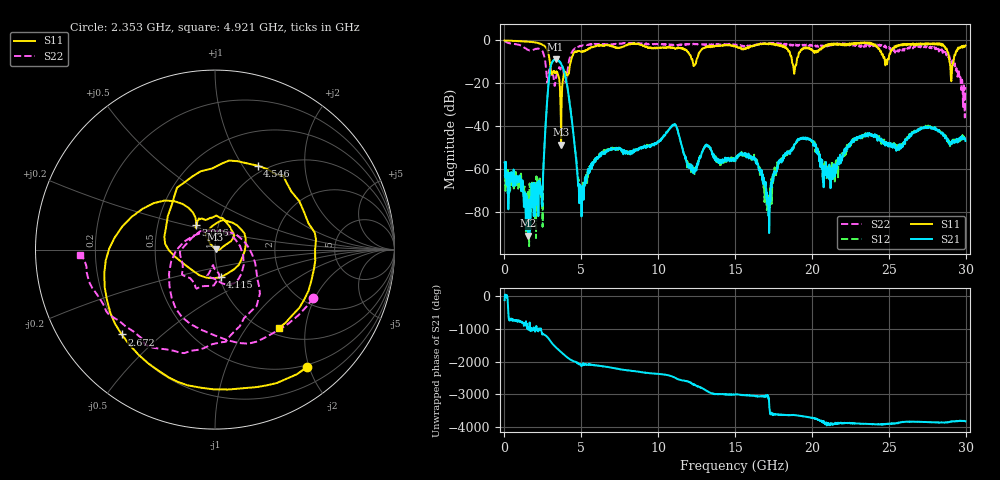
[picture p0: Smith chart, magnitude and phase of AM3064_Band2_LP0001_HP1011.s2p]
# Hz S DB R 50.0
!freq dBS11 angS11 dBS21 angS21 dBS12 angS12 dBS22 angS22
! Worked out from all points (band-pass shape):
!   1600 points, 10 MHz to 29.98 GHz, reference 50 ohm
!   highest |S21| = -8.74 dB at 3.328 GHz (marker M1); lowest = -90.8 dB at 1.528 GHz (marker M2)
!   |S21| within 3 dB of the highest: 3.02 GHz to 3.745 GHz (725.3 MHz wide, 21.4 % of centre)
!   lowest |S11| = -48.5 dB at 3.684 GHz (marker M3), VSWR 1.01, Z = 50.3 + j0.169 ohm
!   |S11| at or under -10 dB: 2.951 GHz to 4.316 GHz (1.365 GHz wide, 37.6 % of centre); 18.71 GHz to 19.01 GHz (297.5 MHz wide, 1.58 % of centre); 28.95 GHz to 29.2 GHz (254.6 MHz wide, 0.876 % of centre)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
!   |S22| runs from -35.8 to -0.2 dB; largest |S21 - S12| = 0.015
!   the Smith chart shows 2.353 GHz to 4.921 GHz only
!   S11 on the Smith chart (normalised r, x): 2.353 GHz: 0.46, -1.96; 2.672 GHz: 0.20, -0.37; 3.046 GHz: 0.78, +0.22; 4.115 GHz: 1.01, -0.32; 4.546 GHz: 0.91, +1.17; 4.921 GHz: 1.12, -1.44
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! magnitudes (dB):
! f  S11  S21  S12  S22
! 10 MHz  0.0  -56.7  -63.1  -0.2
! 1.528 GHz  -0.6  -90.8  -72.5  -4.4
! 2.353 GHz  -1.6  -71.2  -69.6  -4.3
! 2.672 GHz  -3.1  -39.9  -39.9  -10.8
! 3.046 GHz  -15.2  -11.0  -11.0  -15.7
! 3.328 GHz  -15.0  -8.7  -8.9  -18.5
! 3.684 GHz  -48.5  -10.9  -10.8  -12.9
! 4.115 GHz  -16.1  -22.5  -22.6  -13.5
! 4.546 GHz  -5.6  -47.3  -47.2  -4.0
! 4.921 GHz  -5.0  -68.7  -70.8  -2.5
! 5.015 GHz  -5.4  -81.9  -74.8  -2.6
! 6.364 GHz  -2.3  -51.9  -52.0  -1.8
! 10 GHz  -3.4  -46.9  -46.9  -1.7
! 15 GHz  -2.6  -56.0  -56.3  -1.9
! 16.34 GHz  -2.2  -56.5  -55.6  -2.2
! 17.16 GHz  -1.6  -74.0  -72.1  -1.4
! 17.93 GHz  -2.2  -55.5  -56.7  -1.7
! 19.99 GHz  -4.3  -46.8  -46.5  -2.1
! 21.23 GHz  -1.7  -62.2  -58.6  -2.4
! 25 GHz  -8.4  -48.5  -49.2  -3.1
! 28.56 GHz  -2.6  -44.0  -43.4  -5.0
! 29.98 GHz  -2.4  -46.8  -46.7  -21.7
